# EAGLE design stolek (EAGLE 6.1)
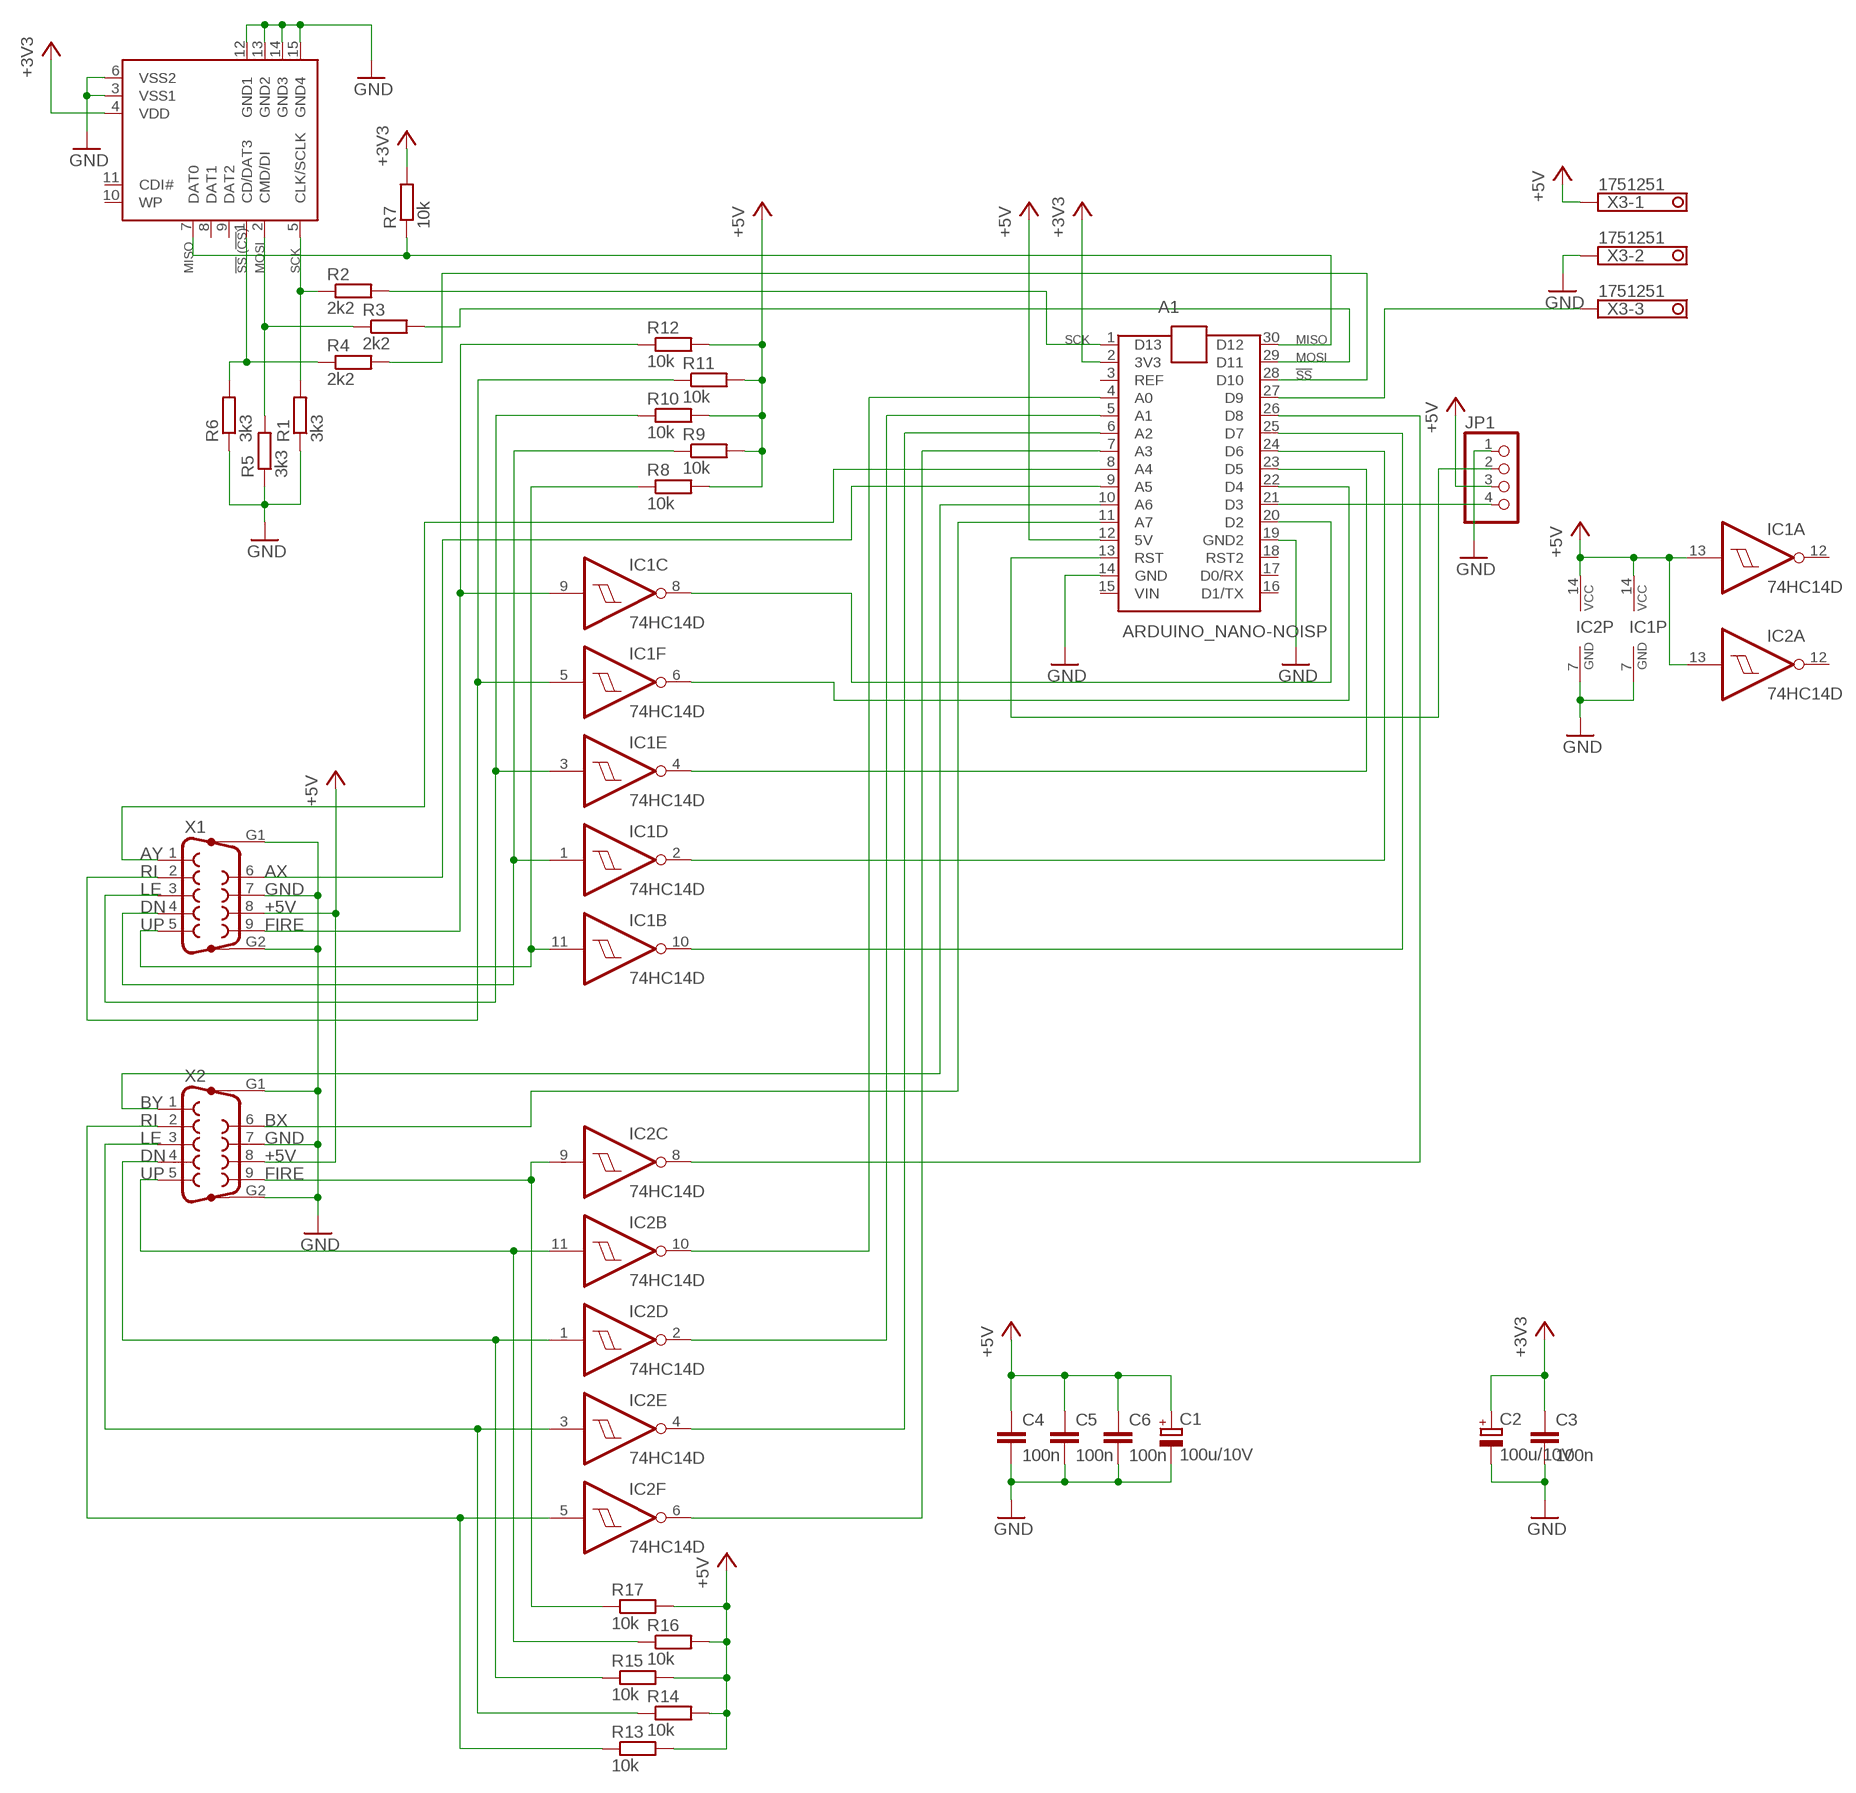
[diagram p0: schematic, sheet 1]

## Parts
A1  ARDUINO_NANO-NOISP  [ARDUINO_NANO_NOISP]
C1  100u/10V  CPOL-EUE2.5-7  [E2,5-7]
C2  100u/10V  CPOL-EUE2.5-7  [E2,5-7]
C3  100n  C-EUC0805  [C0805]
C4  100n  C-EUC0805  [C0805]
C5  100n  C-EUC0805  [C0805]
C6  100n  C-EUC0805  [C0805]
IC1  74HC14D  [SO14]
IC2  74HC14D  [SO14]
JP1  PINHD-1X4-S  [1X04S]
R1  3k3  R-EU_R0805  [R0805]
R2  2k2  R-EU_R0805  [R0805]
R3  2k2  R-EU_R0805  [R0805]
R4  2k2  R-EU_R0805  [R0805]
R5  3k3  R-EU_R0805  [R0805]
R6  3k3  R-EU_R0805  [R0805]
R7  10k  R-EU_R0805  [R0805]
R8  10k  R-EU_R0805  [R0805]
R9  10k  R-EU_R0805  [R0805]
R10  10k  R-EU_R0805  [R0805]
R11  10k  R-EU_R0805  [R0805]
R12  10k  R-EU_R0805  [R0805]
R13  10k  R-EU_R0805  [R0805]
R14  10k  R-EU_R0805  [R0805]
R15  10k  R-EU_R0805  [R0805]
R16  10k  R-EU_R0805  [R0805]
R17  10k  R-EU_R0805  [R0805]
SD1  SLOT-SD030  SDCARDVAR1  [SDCMF-10915W010]
X1  F09HP  [F09HP]
X2  F09HP  [F09HP]
X3  1751251  [1751251]

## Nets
+3V3: A1.2(3V3) C2.+ C3.1 R7.2 SD1.4(VDD)
+5V: A1.12(5V) C1.+ C4.1 C5.1 C6.1 IC1.13(A:I) IC1.14(P:VCC) IC2.13(A:I) IC2.14(P:VCC) JP1.3 R8.2 R9.2 R10.2 R11.2 R12.2 R13.2 R14.2 R15.2 R16.2 R17.2 X1.8 X2.8 X3.1
GND: A1.14(GND) A1.19(GND2) C1.- C2.- C3.2 C4.2 C5.2 C6.2 IC1.7(P:GND) IC2.7(P:GND) JP1.1 R1.1 R5.1 R6.1 SD1.3(VSS1) SD1.6(VSS2) SD1.12(GND1) SD1.13(GND2) SD1.14(GND3) SD1.15(GND4) X1.7 X1.G1 X1.G2 X2.7 X2.G1 X2.G2 X3.2
N$1: IC1.11(B:I) R8.1 X1.5
N$2: IC1.1(D:I) R9.1 X1.4
N$3: IC1.3(E:I) R10.1 X1.3
N$4: IC1.5(F:I) R11.1 X1.2
N$5: IC1.9(C:I) R12.1 X1.9
N$6: R1.2 R2.1 SD1.5(CLK/SCLK)
N$7: R3.1 R5.2 SD1.2(CMD/DI)
N$8: R4.1 R6.2 SD1.1(CD/DAT3)
N$9: A1.28(D10) R4.2
N$10: A1.30(D12) R7.1 SD1.7(DAT0)
N$11: A1.1(D13) R2.2
N$12: A1.29(D11) R3.2
N$13: A1.10(A6) X2.1
N$14: A1.11(A7) X2.6
N$15: IC2.9(C:I) R17.1 X2.9
N$16: IC2.11(B:I) R16.1 X2.5
N$17: IC2.1(D:I) R15.1 X2.4
N$18: IC2.3(E:I) R14.1 X2.3
N$19: IC2.5(F:I) R13.1 X2.2
N$20: A1.20(D2) IC1.8(C:O)
N$21: A1.22(D4) IC1.6(F:O)
N$22: A1.23(D5) IC1.4(E:O)
N$23: A1.24(D6) IC1.2(D:O)
N$24: A1.25(D7) IC1.10(B:O)
N$25: A1.27(D9) X3.3
N$26: A1.26(D8) IC2.8(C:O)
N$27: A1.4(A0) IC2.10(B:O)
N$28: A1.5(A1) IC2.2(D:O)
N$29: A1.6(A2) IC2.4(E:O)
N$30: A1.7(A3) IC2.6(F:O)
N$31: A1.9(A5) X1.6
N$32: A1.8(A4) X1.1
N$33: A1.21(D3) JP1.4
N$34: A1.13(RST) JP1.2
Unconnected: A1.3(REF) A1.16(D1/TX) A1.17(D0/RX) A1.18(RST2) IC1.12(A:O) IC2.12(A:O) SD1.8(DAT1) SD1.9(DAT2) SD1.10(WP) SD1.11(CDI#)

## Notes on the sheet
- MISO | !SS! (!CS!) | MOSI | SCK
- SCK | MISO
- MOSI
- !SS
- AY
- RI | AX
- LE | GND
- DN | +5V
- UP | FIRE
- BY
- RI | BX
- LE | GND
- DN | +5V
- UP | FIRE

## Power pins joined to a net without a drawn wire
VIN: A1.15(VIN)

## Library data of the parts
A1 = jfu_drivers:ARDUINO_NANO-NOISP: Arduino nano no ISP
C1 C2 = rcl:CPOL-EU: POLARIZED CAPACITOR, European symbol
C3-C6 = rcl:C-EU: CAPACITOR, European symbol
IC1 IC2 = 74xx-eu:74*14: Hex schmitt trigger INVERTER
JP1 = pinhead:PINHD-1X4: PIN HEADER
R1-R17 = rcl:R-EU_: RESISTOR, European symbol
SD1 = kingfont_sdcmf10915w010:SDCARD: SD card connector KINGFONT SDCMF-10915W010
X1 X2 = con-subd:F09HP: SUB-D; OC_FARNELL: unknown; OC_NEWARK: unknown
X3 = con-phoenix-350:1751251: MKDS 1/ 3-3,5 Printklemme Nennstrom: 10 A Bemessungsspannung: 160 V Raster: 3,5 mm Polzahl: 3 Montageart: Löten Anschlussart: Schraubanschluss Anschlussrichtung vom Leiter zur Platine: 0° Source: http://eshop.phoenixcontact.com .. 1751251.pdf; OC_FARNELL: unknown; OC_NEWARK: unknown

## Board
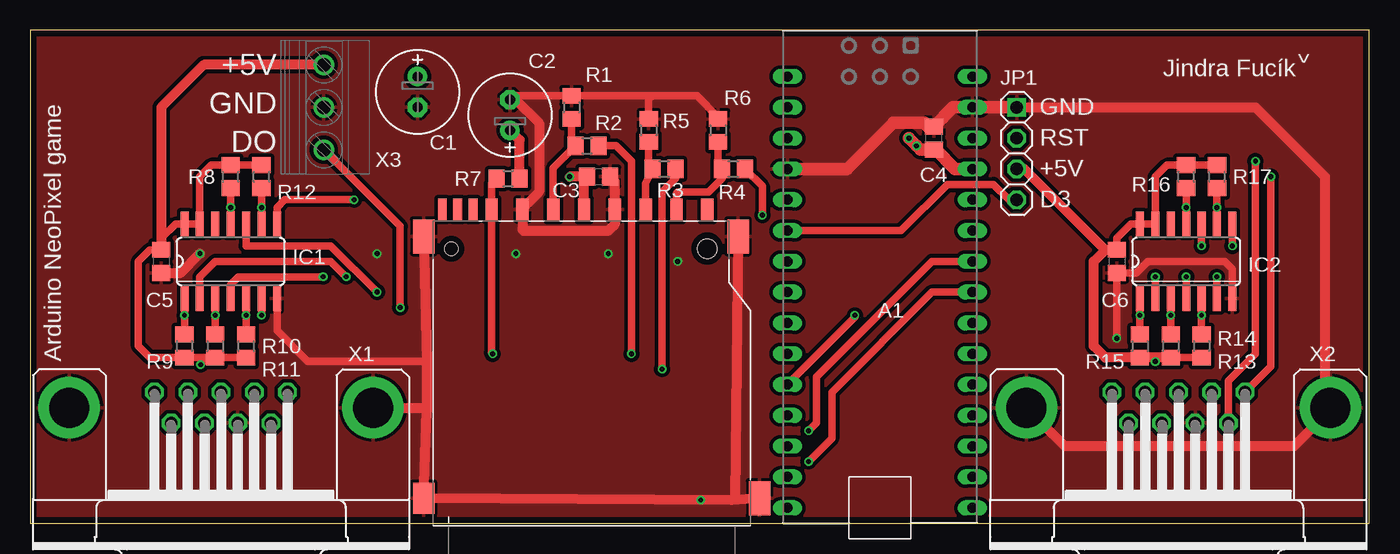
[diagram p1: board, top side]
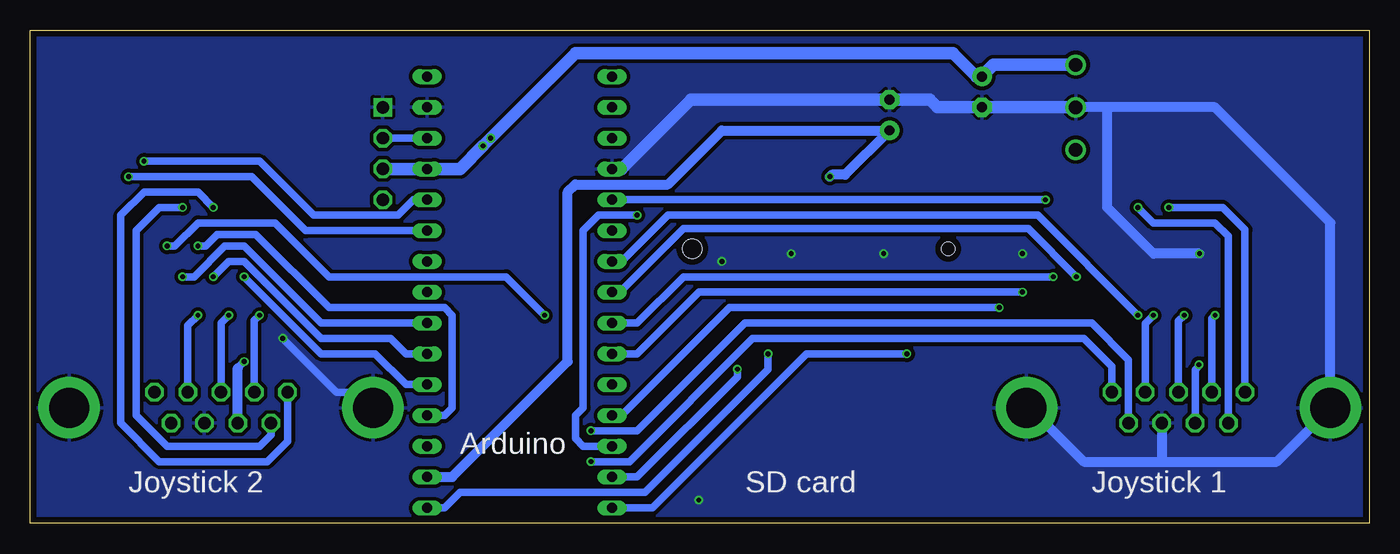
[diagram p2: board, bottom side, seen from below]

Size 110.33 x 40.64 mm. Coordinates in mm from the lower left corner, seen from the top.
Outline: 0,0 110.33,0 110.33,40.64 0,40.64 0,0
Copper layers (1*16): Top 0.035mm / dielectric 1.6mm / Bottom 0.035mm
Design rules: minimum track width 6mil, minimum drill 12mil, track to track 6mil, track to pad 6mil, pad to pad 6mil, via to via 8mil, smd to smd 0mil, copper to edge 20mil, drill to drill 10mil, minimum pad ring 6mil, minimum via ring 6mil, stop-mask expansion 0mil, vias tented up to drill 100mil, thermal gap 10mil

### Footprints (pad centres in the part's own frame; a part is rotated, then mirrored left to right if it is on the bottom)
ARDUINO_NANO_NOISP = drill 0.813 long: 1 -17.78,-7.62; 2 -15.24,-7.62; 3 -12.7,-7.62; 4 -10.16,-7.62; 5 -7.62,-7.62; 6 -5.08,-7.62; 7 -2.54,-7.62; 8 0,-7.62; 9 2.54,-7.62; 10 5.08,-7.62; 11 7.62,-7.62; 12 10.16,-7.62; 13 12.7,-7.62; 14 15.24,-7.62; 15 17.78,-7.62; 16 17.78,7.62; 17 15.24,7.62; 18 12.7,7.62; 19 10.16,7.62; 20 7.62,7.62; 21 5.08,7.62; 22 2.54,7.62; 23 0,7.62; 24 -2.54,7.62; 25 -5.08,7.62; 26 -7.62,7.62; 27 -10.16,7.62; 28 -12.7,7.62; 29 -15.24,7.62; 30 -17.78,7.62
E2,5-7 = drill 0.813 pad 1.6: + -1.27,0 | drill 0.813 pad 1.6 octagon: - 1.27,0
C0805 = smd 1.3 x 1.5: 1 -0.95,0; 2 0.95,0
SO14 = smd 0.66 x 2.032: 1 -3.81,-3.073; 2 -2.54,-3.073; 3 -1.27,-3.073; 4 0,-3.073; 5 1.27,-3.073; 6 2.54,-3.073; 7 3.81,-3.073; 8 3.81,3.073; 9 2.54,3.073; 10 1.27,3.073; 11 0,3.073; 12 -1.27,3.073; 13 -2.54,3.073; 14 -3.81,3.073
1X04S = drill 1.016 square: 1 -3.81,0 | drill 1.016 octagon: 2 -1.27,0; 3 1.27,0; 4 3.81,0
R0805 = smd 1.3 x 1.5: 1 -0.95,0; 2 0.95,0
SDCMF-10915W010 = smd 1.016 x 1.778: 1 7.366,13.64; 2 4.826,13.64; 3 2.286,13.64; 4 -0.254,13.64; 5 -2.794,13.64; 6 -5.334,13.64; 7 -7.874,13.64; 9 9.906,13.64 | smd 0.711 x 1.778: 8 -9.398,13.64; 10 -11.938,13.64; 11 -10.668,13.64 | smd 1.778 x 2.8: 12 12.446,11.43; 13 14.224,-10.16; 15 -13.462,11.43 | smd 1.778 x 2.54: 14 -13.462,-10.16 | hole 1.6: 9.906,10.414 | hole 1.1: -11.176,10.414
F09HP = drill 1.016 octagon: 1 -5.486,-1.27; 2 -2.743,-1.27; 3 0,-1.27; 4 2.743,-1.27; 5 5.486,-1.27; 6 -4.115,1.27; 7 -1.372,1.27; 8 1.372,1.27; 9 4.115,1.27 | drill 3.302 pad 5.08: G1 -12.522,0; G2 12.522,0
1751251 = drill 1.1 pad 1.7: 1 -3.5,-0.1; 2 0,-0.1; 3 3.5,-0.1

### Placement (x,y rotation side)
A1  70.01,19.05 90 top
C1  31.91,35.56 270 top
C2  39.53,33.66 90 top
C3  46.83,28.57 0 top
C4  74.45,31.75 90 top
C5  10.79,21.59 270 top
C6  89.53,21.59 270 top
IC1  16.51,21.59 0 top
IC2  95.25,21.59 0 top
JP1  81.28,30.48 270 top
R1  44.61,34.29 270 top
R2  45.88,31.11 0 top
R3  52.23,29.21 0 top
R4  57.94,29.21 0 top
R5  50.96,32.38 270 top
R6  56.67,32.38 270 top
R7  39.37,28.42 0 top
R8  16.51,28.57 90 top
R9  12.7,14.61 270 top
R10  15.24,14.61 270 top
R11  17.78,14.61 270 top
R12  19.05,28.57 90 top
R13  96.52,14.61 270 top
R14  93.98,14.61 270 top
R15  91.44,14.61 270 top
R16  95.25,28.57 90 top
R17  97.79,28.57 90 top
SD1  45.88,12.22 0 top
X1  15.72,9.53 180 top
X2  94.61,9.53 180 top
X3  24.29,34.29 270 top

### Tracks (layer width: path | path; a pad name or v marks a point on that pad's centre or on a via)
+3V3  (via drill 0.4)
  Top 0.813: R7.2 40.32,31.59 C2.+ | v44.45,28.57 C3.1 45.62,28.32 SD1.4
  Bottom 0.813: v44.45,28.57 44.29,28.73 43.18,28.73 C2.+ 53.34,32.38 57.78,27.94 65.41,27.94 66.04,27.3 66.04,13.34 75.56,3.81 A1.2
+5V  (via drill 0.4)
  Top 0.61: R12.2 R8.2 14.92,29.52 13.97,28.57 IC1.13 IC1.14 11.96,24.66 10.79,23.5 C5.1 9.84,22.54 8.89,21.59 8.89,14.61 9.84,13.65 R9.2 14.61,13.65 | R11.2 R10.2 14.61,13.65 | v14.03,13.08 14.61,13.65 | R13.2 R14.2 | R17.2 R16.2 93.66,29.52 92.71,28.57 IC2.13 IC2.14 90.7,24.66 89.53,23.5 C6.1 88.58,22.54 | v92.71,13.34 92.71,13.65
  Top 0.813: R14.2 92.71,13.65 R15.2 88.58,13.65 87.63,14.61 87.63,21.59 88.58,22.54 81.91,29.21 JP1.3 | X3.1 14.29,37.79 10.79,34.29 C5.1
  Top 1.016: v72.39,31.75 v73.03,31.11 73.34,30.8 C4.1 74.61,30.8 76.2,29.21 A1.12
  Bottom 0.61: v14.03,13.08 14.03,12.96 14.35,12.64 X1.8 | 93.24,12.8 v92.71,13.34
  Bottom 0.813: X2.8 93.24,12.8
  Bottom 1.016: X3.1 30.95,37.79 C1.+ 32.38,36.83 34.29,38.73 65.41,38.73 v73.03,31.11 74.93,29.21 JP1.3
GND  (via drill 0.4)
  Top 0.61: 39.84,35.24 R1.1 51.44,35.24 | R6.1 56.67,33.5 54.93,35.24 51.44,35.24 | R5.1 50.96,35.08 51.44,35.24 | IC2.7 99.06,20.95 98.42,21.59 92.08,21.59 91.12,20.64 C6.2 v89.53,15.24 | IC1.7 20.32,15.88 22.86,13.34 32.67,13.34
  Top 0.813: C3.2 48.16,28.19 SD1.3 48.16,24.67 47.62,24.13 40.64,24.13 40.55,24.23 SD1.6 40.55,25.94 41.91,27.3 41.91,33.02 40.01,34.92 C2.- 39.84,35.24 | C5.2 12.38,20.64 v13.97,22.23 | X1.G1 32.38,9.53 32.67,9.24 | 32.67,9.24 SD1.14 57.78,1.91 | SD1.15 32.67,13.34 32.67,9.24 | SD1.13 57.78,1.91 | SD1.12 58.07,2.19 57.78,1.91 | 95.89,6.35 104.14,6.35 107.14,9.35 X2.G1 106.68,9.98 106.68,28.57 100.97,34.29 JP1.1 | 95.89,6.35 85.27,6.35 X2.G2 | X2.7 95.99,6.45 95.89,6.35
  Top 1.016: A1.19 67.31,29.21 71.12,33.02 73.66,33.02 73.98,32.7 C4.2 76.04,34.29 A1.14 JP1.1
  Bottom 0.61: v89.53,15.24 85.09,10.79 83.36,10.79 X2.G2
  Bottom 0.813: v13.97,22.23 17.78,22.23 21.59,26.04 21.59,34.29 | 21.59,34.29 12.7,34.29 3.19,24.78 X1.G2 3.17,9.53 7.62,5.08 17.14,5.08 | 21.59,34.29 X3.2 | X1.G1 27.94,9.53 23.5,5.08 17.14,5.08 | X1.7 17.09,5.14 17.14,5.08
  Bottom 1.016: X3.2 C1.- 35.56,34.29 36.2,34.92 C2.- 55.88,34.92 61.59,29.21 A1.19
  other vias: 55.24,1.91 40.01,22.23 47.62,22.23 28.57,22.23 53.34,21.59
  pour Top (isolate 0.305): 110.49,40.64 0,40.64 0,0 110.49,0
  pour Bottom (isolate 0.305): 0,0 110.49,0 110.49,40.64 0,40.64
N$1  (via drill 0.4)
  Top 0.61: R8.1 v16.51,26.04 IC1.11
  Bottom 0.61: X1.5 10.23,24.2 12.06,26.04 v16.51,26.04
N$2  (via drill 0.4)
  Top 0.61: R9.1 v12.7,17.14 IC1.1
  Bottom 0.61: X1.4 12.97,16.87 v12.7,17.14
N$3  (via drill 0.4)
  Top 0.61: R10.1 v15.24,17.14 IC1.3
  Bottom 0.61: X1.3 15.72,16.67 v15.24,17.14
N$4  (via drill 0.4)
  Top 0.61: R11.1 v17.78,17.14 IC1.5
  Bottom 0.61: X1.2 18.46,16.47 v17.78,17.14
N$5  (via drill 0.4)
  Top 0.61: R12.1 v19.05,26.04 IC1.9
  Bottom 0.61: X1.9 11.6,23.67 12.7,24.77 17.78,24.77 v19.05,26.04
N$6
  Top 0.61: SD1.5 43.09,29.27 R2.1 44.61,31.43 R1.2
N$7
  Top 0.61: SD1.2 50.7,28 R3.1 50.96,29.53 R5.2
N$8
  Top 0.61: R6.2 56.67,29.53 R4.1 56.99,28.42 55.88,27.3 53.34,27.3 53.24,27.21 SD1.1
N$9  (via drill 0.4)
  Top 0.61: R4.2 60.33,27.78 v60.33,25.4
  Bottom 0.61: v60.33,25.4 63.5,25.4 64.77,24.13 64.77,9.53 65.41,8.89 65.41,6.99 64.77,6.35 A1.28
N$10  (via drill 0.4)
  Top 0.61: R7.1 38.01,28 SD1.7 38.01,14.06 v38.1,13.97
  Bottom 0.61: A1.30 59.05,1.27 46.35,13.97 v38.1,13.97
N$11  (via drill 0.4)
  Top 0.61: R2.2 48.26,31.11 49.53,29.84 v49.53,13.97
  Bottom 0.61: v49.53,13.97 49.53,12.7 59.69,2.54 74.93,2.54 76.2,1.27 A1.1
N$12  (via drill 0.4)
  Top 0.61: R3.2 53.18,28.41 52.07,27.3 v52.07,12.7
  Bottom 0.61: v52.07,12.7 52.07,12.06 60.33,3.81 A1.29
N$13  (via drill 0.4)
  Top 0.61: v102.23,28.57 102.23,12.93 X2.1
  Bottom 0.61: A1.10 87.63,24.13 92.08,28.57 v102.23,28.57
N$14  (via drill 0.4)
  Top 0.61: v100.97,29.84 100.97,13.97 98.73,11.73 X2.6
  Bottom 0.61: A1.11 78.74,26.67 80.01,25.4 87,25.4 91.44,29.84 v100.97,29.84
N$15  (via drill 0.4)
  Top 0.61: R17.1 v97.79,26.04 IC2.9
  Bottom 0.61: X2.9 90.5,7.29 91.44,6.35 99.06,6.35 101.6,8.89 101.6,24.13 99.69,26.04 v97.79,26.04
N$16  (via drill 0.4)
  Top 0.61: R16.1 v95.25,26.04 IC2.11
  Bottom 0.61: X2.5 89.13,6.76 90.81,5.08 99.69,5.08 102.87,8.26 102.87,25.4 100.97,27.3 96.52,27.3 v95.25,26.04
N$17  (via drill 0.4)
  Top 0.61: IC2.1 91.44,17.78 v91.44,17.14 R15.1
  Bottom 0.61: X2.4 91.87,16.71 v91.44,17.14
N$18  (via drill 0.4)
  Top 0.61: IC2.3 93.98,17.78 v93.98,17.14 R14.1
  Bottom 0.61: X2.3 94.61,16.51 v93.98,17.14
N$19  (via drill 0.4)
  Top 0.61: IC2.5 96.52,17.78 v96.52,17.14 R13.1
  Bottom 0.61: X2.2 97.36,16.31 v96.52,17.14
N$20  (via drill 0.4)
  Top 0.61: IC1.8 20.32,26.04 20.95,26.67 v26.67,26.67
  Bottom 0.61: A1.20 v26.67,26.67
N$21  (via drill 0.4)
  Top 0.61: v19.05,17.14 IC1.6
  Bottom 0.61: A1.22 61.59,21.59 57.78,25.4 27.3,25.4 v19.05,17.14
N$22  (via drill 0.4)
  Top 0.61: v24.13,20.32 17.14,20.32 16.51,19.68 IC1.4 16.51,18.41
  Bottom 0.61: A1.23 61.75,19.05 56.52,24.29 28.1,24.29 v24.13,20.32
N$23  (via drill 0.4)
  Top 0.61: v26.04,20.32 24.77,21.59 15.24,21.59 13.97,20.32 IC1.2
  Bottom 0.61: A1.24 60.33,16.51 56.52,20.32 v26.04,20.32
N$24  (via drill 0.4)
  Top 0.61: IC1.10 17.78,22.86 24.77,22.86 v28.57,19.05
  Bottom 0.61: v28.57,19.05 55.24,19.05 60.33,13.97 A1.25
N$25  (via drill 0.4)
  Top 0.61: v30.48,17.78 30.48,24.5 X3.3
  Bottom 0.61: A1.27 61.59,8.89 52.7,17.78 v30.48,17.78
N$26  (via drill 0.4)
  Top 0.61: IC2.8 v99.06,22.86 | v67.94,17.14 67.94,16.99 A1.26
  Bottom 0.61: v99.06,22.86 98.42,22.86 96.52,24.77 90.17,24.77 85.72,20.32 71.12,20.32 v67.94,17.14
N$27  (via drill 0.4)
  Top 0.61: IC2.10 v96.52,22.86
  Bottom 0.61: v96.52,22.86 95.89,22.86 94.93,23.81 91.76,23.81 85.72,17.78 76.2,17.78 75.56,17.14 75.56,9.53 76.2,8.89 A1.4
N$28  (via drill 0.4)
  Top 0.61: IC2.2 v92.71,20.32
  Bottom 0.61: v92.71,20.32 86.36,13.97 81.92,13.97 79.38,11.43 A1.5
N$29  (via drill 0.4)
  Top 0.61: IC2.4 v95.25,20.32
  Bottom 0.61: v95.25,20.32 93.98,21.59 92.71,21.59 86.36,15.24 80.64,15.24 79.38,13.97 A1.6
N$30  (via drill 0.4)
  Top 0.61: IC2.6 v97.79,20.32
  Bottom 0.61: v97.79,20.32 96.84,20.32 94.3,22.86 92.71,22.86 86.36,16.51 A1.7
N$31  (via drill 0.4)
  Top 0.61: A1.9 74.3,21.59 64.77,12.06 64.77,8.26 v64.14,7.62
  Bottom 0.61: v64.14,7.62 60.33,7.62 51.44,16.51 22.86,16.51 19.83,13.48 X1.6
N$32  (via drill 0.4)
  Top 0.61: A1.8 74.3,19.05 66.04,10.79 66.04,6.99 v64.14,5.08
  Bottom 0.61: v64.14,5.08 60.96,5.08 50.8,15.24 23.5,15.24 21.2,12.95 X1.1
N$33
  Top 0.61: A1.21 71.75,24.13 75.56,27.94 79.38,27.94 80.64,26.67 JP1.4
N$34
  Bottom 0.61: A1.13 JP1.2

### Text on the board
tPlace: +5V | ^ | Jindra Fucík | GND | GND | DO | RST | +5V | D3 | Arduino NeoPixel game
bPlace: Arduino | Joystick 1 | SD card | Joystick 2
